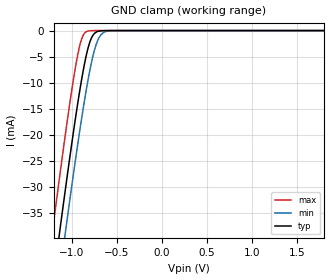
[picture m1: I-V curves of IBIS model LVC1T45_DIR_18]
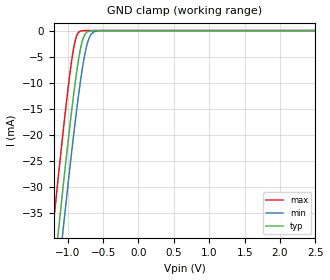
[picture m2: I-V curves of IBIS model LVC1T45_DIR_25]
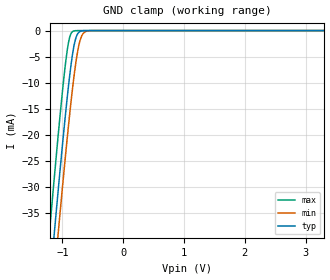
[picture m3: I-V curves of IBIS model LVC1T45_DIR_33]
| TEXAS INSTRUMENTS INCORPORATED
| IBIS Model of SN74LVC1T45
| Single-Bit Dual Supply Bus Transceiver with Configurable Output Voltage
| Translation and 3-State Outputs
| This file contains package information for the following:
|  SOT 6-pin (DBV) package as [Component] LVC1T45_DBV
|  DSBGA 6-pin (YEP_YZP) package as [Component] LVC1T45_YEP_YZP
|  SOT 6-pin (DCK) package as [Component] LVC1T45_DCK
| This device can be powered at the following Vccs:
|  1.8 volt Vcc
|  2.5 volt Vcc
|  3.3 volt Vcc
|  5 volt Vcc
|  2.8 volt Vcc
| This file provides unique models under the [Model Selector] for each Vcc.
| For operation at a specific Vcc, select the appropriate model after each
| [Model Selector] keyword.
[IBIS Ver]   4.1
[Comment char]  |_char
[File Name]   sn74lvc1t45.ibs
[File Rev]   1.4 | x_die
[Date]   January 08, 2015
[Source]   Data created from TI-SPICE simulations at TI-SLL.
   Texas Instruments Incorporated.
   Analog-eLab, HPA
   12500 TI Blvd
   Dallas, TX -75243
   For Support e-mail: elab_ibis@list.ti.com
[Notes]   The following is an IBIS list for the SN74LVC1T45.
   - FILE REV HISTORY
   - 1.1 Release IBIS file on 09/29/03
   - 1.2 YEP and YZP packages released on 04/30/04
   - 1.3 Added 2.8 V voltage range  05/24/06
   - Power clamp data deleted as there is no power-clamp diode.
   - Due to the fact that the Device is 5-V Input/Output
   tolarent, the pulldown has some Non-Monotonic Warnings.
   - 1.4 Added DRL package component on 1/8/15
[Disclaimer]  This model is designed as an aid for customers of Texas Instruments
 TI and its licensors and suppliers make no warranties, either expressed
 or implied, with respect to this  model, including the warranties of
 merchantability or fitness for a particular purpose.
 The model is provided solely on an "as is" basis. The entire risk as to
 its quality and performance is with the customer.
[Copyright] (C)Copyright 2014 Texas Instruments Incorporated.
   All rights reserved.
| Component SN74LVC1T45_DBV 6-PIN SOT
[Component]   SN74LVC1T45_DBV
[Manufacturer]   Texas Instruments, Inc.
[Package]
|   typ   min   max
R_pkg   2.500e-02   1.900e-02   3.700e-02
L_pkg   1.524e-09   1.260e-09   1.751e-09
C_pkg   2.450e-13   1.980e-13   2.640e-13
[Pin]   signal_name   model_name   R_pin   L_pin   C_pin
1   VCCA   POWER   2.100e-02   1.405e-09   2.460e-13
2   GND   GND   3.700e-02   1.751e-09   2.630e-13
3   A   LVC1T45_IO_A   2.600e-02   1.493e-09   2.470e-13
4   B   LVC1T45_IO_B   1.900e-02   1.620e-09   2.640e-13
5   DIR   LVC1T45_DIR   2.400e-02   1.260e-09   1.980e-13
6   VCCB   POWER   2.100e-02   1.617e-09   2.500e-13
| Component SN74LVC1T45_DCK 6-PIN SOT
[Component]   SN74LVC1T45_DCK
[Manufacturer]   Texas Instruments, Inc.
[Package]
|   typ   min   max
R_pkg   1.400e-02   1.100e-02   2.100e-02
L_pkg   9.480e-10   7.840e-10   1.103e-09
C_pkg   1.910e-13   1.670e-13   2.050e-13
[Pin]   signal_name   model_name   R_pin   L_pin   C_pin
1   VCCA   POWER   1.300e-02   9.840e-10   1.960e-13
2   GND   GND   2.100e-02   1.103e-09   2.050e-13
3   A   LVC1T45_IO_A   1.100e-02   9.980e-10   1.970e-13
4   B   LVC1T45_IO_B   1.300e-02   9.040e-10   1.900e-13
5   DIR   LVC1T45_DIR   1.500e-02   7.840e-10   1.670e-13
6   VCCB   POWER   1.200e-02   9.160e-10   1.950e-13
| Component SN74LVC1T45_YEP_YZP 6-PIN DSBGA
[Component]   SN74LVC1T45_YEP_YZP
[Manufacturer]   Texas Instruments, Inc.
[Package]
|   typ   min   max
R_pkg   1.000e-03   1.000e-03   4.000e-03
L_pkg   7.500e-11   2.400e-11   3.790e-10
C_pkg   5.600e-14   0.000e+00   6.700e-14
[Pin]   signal_name   model_name   R_pin   L_pin   C_pin
1   VCCA   POWER   1.000e-03   2.500e-11   6.400e-14
2   GND   GND   1.000e-03   2.400e-11   6.700e-14
3   A   LVC1T45_IO_A   1.000e-03   2.500e-11   6.400e-14
4   B   LVC1T45_IO_B   1.000e-03   2.500e-11   6.400e-14
5   DIR   LVC1T45_DIR   1.000e-03   2.400e-11   6.700e-14
6   VCCB   POWER   1.000e-03   2.500e-11   6.400e-14
| Component SN74LVC1T45_DRL 6-PIN SOT
[Component]   SN74LVC1T45_DRL
[Manufacturer]   Texas Instruments, Inc.
[Package]
|   typ   min   max
R_pkg   0.03671   0.03637   0.03748
L_pkg   0.66545n   0.36880n   0.73034n
C_pkg   0.12310p   0.10158p   0.13769p
[Pin]   signal_name   model_name   R_pin   L_pin   C_pin
1   VCCA   POWER   0.03748   0.56880n   0.10158p
2   GND   GND   0.03674   0.73034n   0.13769p
3   A   LVC1T45_IO_A   0.03647   0.68968n   0.12163p
4   B   LVC1T45_IO_B   0.03637   0.58388n   0.11837p
5   DIR   LVC1T45_DIR   0.03647   0.68968n   0.12163p
6   VCCB   POWER   0.03674   0.73034n   0.13769p
| Model LVC1T45_DIR
[Model Selector]   LVC1T45_DIR
LVC1T45_DIR_18   1.8 volt Vcc
LVC1T45_DIR_25   2.5 volt Vcc
LVC1T45_DIR_33   3.3 volt Vcc
LVC1T45_DIR_50   5 volt Vcc
LVC1T45_DIR_28A   2.8 volt Vcc
| Model LVC1T45_IO_B
[Model Selector]   LVC1T45_IO_B
LVC1T45_IO_B_18   1.8 volt Vcc
LVC1T45_IO_B_25   2.5 volt Vcc
LVC1T45_IO_B_33   3.3 volt Vcc
LVC1T45_IO_B_50   5 volt Vcc
LVC1T45_IO_B_28A   2.8 volt Vcc
| Model LVC1T45_IO_A
[Model Selector]   LVC1T45_IO_A
LVC1T45_IO_A_18   1.8 volt Vcc
LVC1T45_IO_A_25   2.5 volt Vcc
LVC1T45_IO_A_33   3.3 volt Vcc
LVC1T45_IO_A_50   5 volt Vcc
LVC1T45_IO_A_28A   2.8 volt Vcc
| Models and submodels in the file (15): LVC1T45_DIR_18 (Input), LVC1T45_DIR_25 (Input), LVC1T45_DIR_33 (Input), LVC1T45_DIR_50 (Input), LVC1T45_DIR_28A (Input), LVC1T45_IO_B_18 (I/O), LVC1T45_IO_B_25 (I/O), LVC1T45_IO_B_33 (I/O), LVC1T45_IO_B_50 (I/O), LVC1T45_IO_B_28A (I/O), LVC1T45_IO_A_18 (I/O), LVC1T45_IO_A_25 (I/O), LVC1T45_IO_A_33 (I/O), LVC1T45_IO_A_50 (I/O), LVC1T45_IO_A_28A (I/O)
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[Model]   LVC1T45_DIR_18
Model_type  Input
Vinl=0.5775
Vinh=1.2675
| variable   typ   min   max
C_comp   3.23pF   2.70pF   4.14pF
[Temperature Range]   40   100   -40
| Ambient temperature   25   85   -40
[Voltage range]   1.8   1.65   1.95
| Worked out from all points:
|   GND clamp passes 1 mA (typ) near -0.77 V on its own axis
[GND Clamp]
| LVC1T45_DIR_18
|   Voltage   I(typ)   I(min)   I(max)
-5.5V     -655.2mA   -662.2mA   -646.6mA
-1.215V   -49.6mA    -57.88mA   -38.96mA
-1.135V   -39.07mA   -47.36mA   -28.42mA
-1.075V   -31.35mA   -39.6mA    -20.75mA
-1.055V   -28.82mA   -37.05mA   -18.27mA
-955mV    -16.68mA   -24.66mA   -6.874mA
-885mV    -9.098mA   -16.55mA   -1.486mA
-825mV    -3.922mA   -10.26mA   -137.1uA
-780mV    -1.472mA   -6.227mA   -17.15uA
-715mV    -205.4uA   -2.128mA   -808.5nA
-650mV    -22.01uA   -443.9uA   -37.93nA
1.8V      3.326pA    6.142pA    3.026pA
[Model]   LVC1T45_DIR_25
Model_type  Input
Vinl=0.7
Vinh=1.7
| variable   typ   min   max
C_comp   3.14pF   2.55pF   4.16pF
[Temperature Range]   40   100   -40
| Ambient temperature   25   85   -40
[Voltage range]   2.5   2.3   2.7
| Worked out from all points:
|   GND clamp passes 1 mA (typ) near -0.77 V on its own axis
[GND Clamp]
| LVC1T45_DIR_25
|   Voltage   I(typ)   I(min)   I(max)
-5.5V     -655.2mA   -662.2mA   -646.6mA
-1.215V   -49.6mA    -57.88mA   -38.96mA
-1.14V    -39.72mA   -48.01mA   -29.07mA
-1.12V    -37.12mA   -45.41mA   -26.48mA
-1.08V    -31.98mA   -40.25mA   -21.38mA
-1.06V    -29.44mA   -37.69mA   -18.89mA
-960mV    -17.26mA   -25.26mA   -7.377mA
-890mV    -9.597mA   -17.1mA    -1.734mA
-785mV    -1.671mA   -6.635mA   -21.67uA
-720mV    -242.5uA   -2.354mA   -1.023uA
-650mV    -22.01uA   -443.9uA   -37.93nA
2.5V      4.713pA    7.577pA    4.389pA
[Model]   LVC1T45_DIR_33
Model_type  Input
Vinl=0.8
Vinh=2.0
| variable   typ   min   max
C_comp   3.06pF   2.42pF   4.23pF
[Temperature Range]   40   100   -40
| Ambient temperature   25   85   -40
[Voltage range]   3.3   3   3.6
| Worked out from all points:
|   GND clamp passes 1 mA (typ) near -0.77 V on its own axis
[GND Clamp]
| LVC1T45_DIR_33
|   Voltage   I(typ)   I(min)   I(max)
-5.5V     -655.2mA   -662.2mA   -646.6mA
-1.225V   -50.93mA   -59.21mA   -40.3mA
-1.145V   -40.37mA   -48.66mA   -29.72mA
-1.12V    -37.12mA   -45.41mA   -26.48mA
-1.08V    -31.98mA   -40.25mA   -21.38mA
-1.06V    -29.44mA   -37.69mA   -18.89mA
-965mV    -17.84mA   -25.87mA   -7.89mA
-885mV    -9.098mA   -16.55mA   -1.486mA
-780mV    -1.472mA   -6.227mA   -17.15uA
-715mV    -205.4uA   -2.128mA   -808.5nA
-640mV    -15.53uA   -338.1uA   -23.69nA
3.3V      6.304pA    9.258pA    5.93pA
